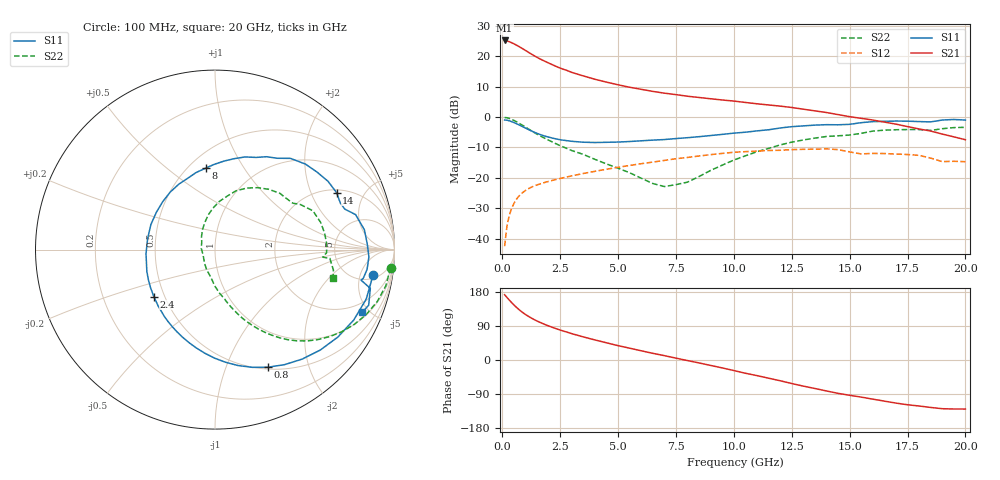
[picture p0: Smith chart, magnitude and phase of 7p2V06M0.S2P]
! Infineon Technologies  Discrete & RF Semiconductors
! bfp620
! VCE =  2.0 V,  IC =  6.0 mA
! Common Emitter S-Parameters:  Sep 2002
# GHz  S  MA  R  50
!  f  S11  S21  S12  S22
! GHz  MAG  ANG  MAG  ANG  MAG  ANG  MAG  ANG
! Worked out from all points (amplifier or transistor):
!   59 points, 100 MHz to 20 GHz, reference 50 ohm
!   highest |S21| = 25.2 dB at 100 MHz (marker M1)
!   |S21| within 3 dB of that: start of sweep to 940.9 MHz
!   unconditionally stable (mu >= 1): 4.6 GHz to 11.48 GHz; 14.84 GHz to 15.17 GHz; 17.15 GHz to end of sweep
!   at 1 GHz: K = 0.36, MSG = 23.0 dB, |S12| = -24.2 dB
!   at 5.5 GHz: K = 1.05, MAG = 11.6 dB, |S12| = -15.9 dB
!   at 20 GHz: K = 1.33, MAG = 0.2 dB, |S12| = -14.7 dB
!   S11 on the Smith chart (normalised r, x): 100 MHz: 6, -8; 800 MHz: 0.52, -1.41; 2.4 GHz: 0.44, -0.28; 8 GHz: 0.60, +0.69; 14 GHz: 2.15, +3.10; 20 GHz: 1.33, -4.52
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0.1  0.8923 -9.0  18.18 172.3  0.0075 77.8  0.9836 -5.9
0.2  0.8865 -18.1  17.86 165.2  0.016 78.5  0.9729 -12.0
0.3  0.8669 -26.9  17.34 158.3  0.0239 75.0  0.949 -17.8
0.4  0.8404 -35.4  16.71 151.7  0.0311 71.1  0.917 -23.2
0.5  0.8109 -43.6  16.03 145.5  0.0377 67.3  0.8803 -28.3
0.6  0.7802 -51.4  15.32 139.6  0.0437 63.7  0.8411 -33.0
0.8  0.7185 -65.8  13.87 129.1  0.0538 57.5  0.7606 -41.3
1.1  0.6307 -84.6  11.8 116.3  0.0653 50.3  0.6461 -51.0
1.3  0.5801 -95.6  10.6 109.2  0.0713 46.7  0.5795 -55.9
1.5  0.5382 -105.6  9.595 102.9  0.0763 43.9  0.5227 -60.0
1.9  0.4784 -123.2  8.061 92.3  0.0852 39.9  0.4343 -66.5
2.4  0.43 -142.4  6.61 81.1  0.0955 36.2  0.3514 -72.8
3  0.3984 -162.4  5.424 69.5  0.1076 32.5  0.2807 -79.0
3.5  0.385 -176.6  4.742 60.9  0.1178 29.6  0.2425 -84.3
5  0.3873 147.4  3.388 37.9  0.1489 20.3  0.1439 -102.2
7  0.4257 110.8  2.469 11.5  0.1932 6.1  0.0718 -159.7
8  0.4568 96.6  2.197 -1.5  0.2161 -2.6  0.0849 150.3
10.5  0.5622 66.0  1.736 -35.0  0.2693 -28.0  0.23 93.1
13.5  0.7358 31.1  1.262 -75.2  0.2957 -59.7  0.4495 48.4
14  0.7481 25.1  1.186 -81.7  0.2994 -66.1  0.4782 41.1
17  0.8584 -2.7  0.764 -113.7  0.246 -90.5  0.6173 8.7
20  0.8913 -23.1  0.423 -129.4  0.184 -103.6  0.6762 -13.3
